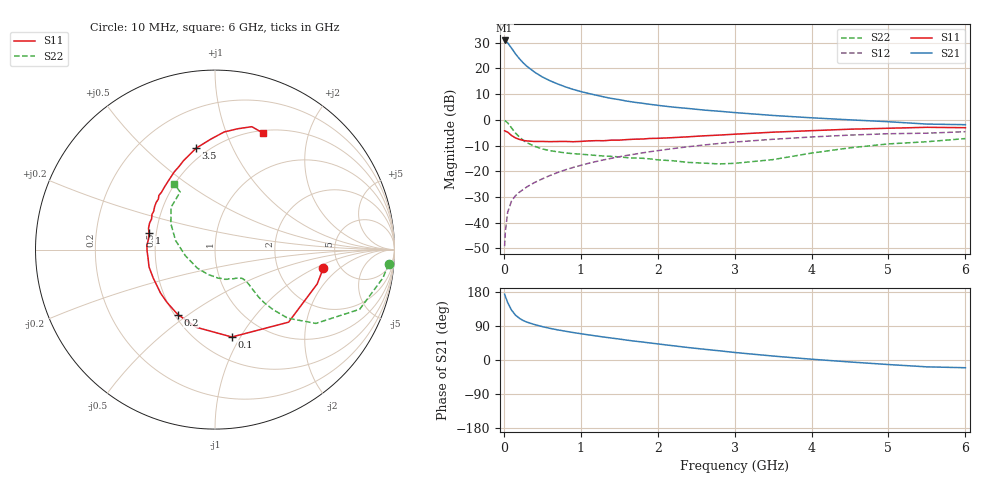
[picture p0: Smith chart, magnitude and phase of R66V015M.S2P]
! SIEMENS Small Signal Semiconductors
! BFR193
! Si NPN RF Bipolar Junction Transistor in SOT23
! VCE = 6 V  IC = 15 mA
! Common Emitter S-Parameters:  May  1996
# GHz  S  MA  R  50
!  f  S11  S21  S12  S22
! GHz  MAG  ANG  MAG  ANG  MAG  ANG  MAG  ANG
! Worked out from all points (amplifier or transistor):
!   36 points, 10 MHz to 6 GHz, reference 50 ohm
!   highest |S21| = 30.8 dB at 10 MHz (marker M1)
!   |S21| within 3 dB of that: start of sweep to 100.5 MHz
!   unconditionally stable (mu >= 1): 667.5 MHz to 1.899 GHz; 1.905 GHz to 2.043 GHz
!   at 250 MHz: K = 0.75, MSG = 24.6 dB, |S12| = -27.1 dB
!   at 1.4 GHz: K = 1.03, MAG = 10.6 dB, |S12| = -15.0 dB
!   at 6 GHz: K = 0.94, MSG = 1.4 dB, |S12| = -4.6 dB
!   S11 on the Smith chart (normalised r, x): 10 MHz: 3.73, -1.22; 100 MHz: 0.71, -0.92; 200 MHz: 0.52, -0.46; 1 GHz: 0.45, +0.10; 3.5 GHz: 0.43, +0.73; 6 GHz: 0.53, +1.35
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0.01  0.6125 -9.6  34.86 173.7  0.0035 82.1  0.9707 -4.8
0.02  0.6006 -18.6  34.18 167.6  0.0068 82.2  0.9487 -9.6
0.05  0.5758 -44.6  31.28 151.6  0.016 73.9  0.8721 -22.4
0.1  0.4959 -79.1  24.74 131.7  0.0264 63.2  0.6963 -36.2
0.15  0.4452 -103.5  19.24 118.7  0.0333 59.7  0.5571 -43.3
0.2  0.4171 -119.8  15.55 110.4  0.039 59.6  0.4672 -45.9
0.25  0.3975 -132.4  12.86 104.3  0.0441 60.3  0.4023 -47.2
0.3  0.3883 -141.4  10.96 99.9  0.0497 61.5  0.3587 -47.4
0.4  0.3789 -155.4  8.44 93.5  0.0605 63.5  0.3055 -46.6
0.5  0.38 -165.2  6.811 88.1  0.0712 65.3  0.2721 -45.8
0.6  0.3761 -172.2  5.745 83.5  0.0827 65.7  0.2513 -45.5
0.7  0.3787 -179.1  4.977 79.5  0.0946 66.5  0.2385 -45.7
0.8  0.3797 176.1  4.371 76.0  0.1067 66.2  0.2274 -46.2
1  0.3803 165.6  3.543 69.4  0.1302 65.4  0.2148 -48.0
1.1  0.3891 162.1  3.258 66.4  0.1427 65.0  0.2089 -50.1
1.3  0.3924 154.2  2.788 60.6  0.1668 63.5  0.1978 -53.7
1.6  0.4128 144.6  2.31 52.4  0.2035 60.5  0.1839 -61.8
2.2  0.4506 128.1  1.765 37.6  0.276 53.6  0.16 -83.7
3.5  0.575 100.5  1.215 10.4  0.4186 34.9  0.1685 -168.3
4.5  0.6571 85.6  0.998 -5.2  0.5046 20.5  0.2856 149.5
5.5  0.7149 73.3  0.826 -18.1  0.5497 5.8  0.3749 121.2
6  0.7026 67.8  0.804 -20.4  0.5874 1.6  0.4318 121.7
